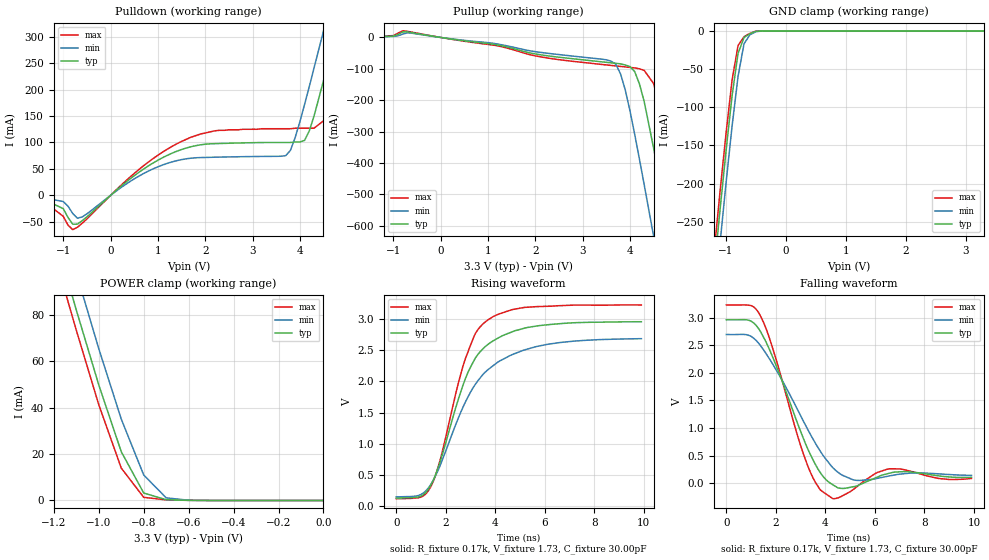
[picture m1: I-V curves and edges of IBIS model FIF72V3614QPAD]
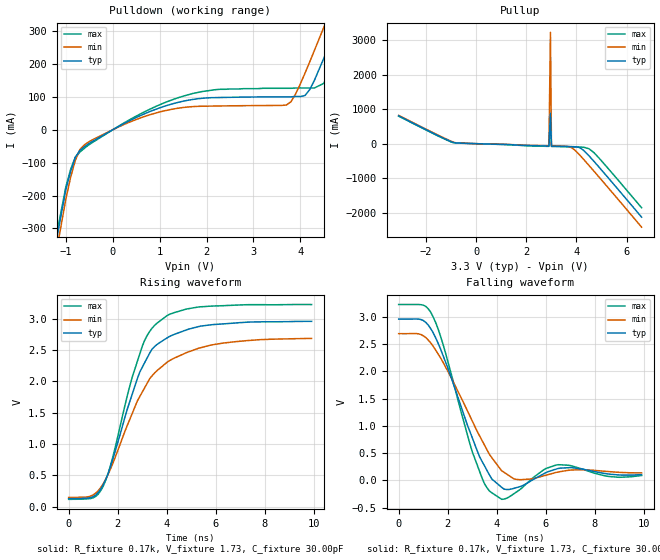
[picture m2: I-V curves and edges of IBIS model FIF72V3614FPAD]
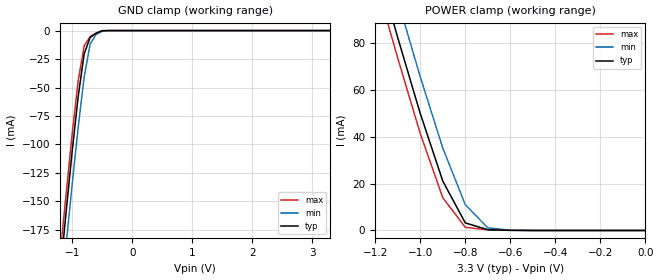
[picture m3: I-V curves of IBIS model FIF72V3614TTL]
| IBIS file i72v3612.ibs created by s2ibis2 version 1.1
| North Carolina State University Electronics Research Laboratory  1995
[IBIS ver]   2.1
[File name]   i72v3612.ibs
[File Rev]   1.0
[Date]   05/01/98
[Source]   Integrated Device Technology, Inc.
[Notes]   1. Temperatures: typ=25C, min=70C, max=0C 2. Cemos8_3.3V
   process. 3. Ramp rates based on 50 ohm load.
[Copyright]   Copyright 1997, Integrated Device Technology, Inc.
|   Component idt72V3612
[Component]   idt72V3612
[Manufacturer]   Integrated Device Technology
[Package]
| variable   typ   min   max
R_pkg   0.75   0.60   0.90
L_pkg   8.10nH   8.30nH   9.90nH
C_pkg   0.53pF   0.46pF   0.60pF
[Pin]  signal_name   model_name   R_pin   L_pin   C_pin
1   A23   FIF72V3614QPAD
2   A22   FIF72V3614QPAD
3   A21   FIF72V3614QPAD
4   GND   GND
5   A20   FIF72V3614QPAD
6   A19   FIF72V3614QPAD
7   A18   FIF72V3614QPAD
8   A17   FIF72V3614QPAD
9   A16   FIF72V3614QPAD
10   A15   FIF72V3614QPAD
11   A14   FIF72V3614QPAD
12   A13   FIF72V3614QPAD
13   A12   FIF72V3614QPAD
14   A11   FIF72V3614QPAD
15   A10   FIF72V3614QPAD
16   GND   GND
17   A9   FIF72V3614QPAD
18   A8   FIF72V3614QPAD
19   A7   FIF72V3614QPAD
20   VCC   POWER
21   A6   FIF72V3614QPAD
22   A5   FIF72V3614QPAD
23   A4   FIF72V3614QPAD
24   A3   FIF72V3614QPAD
25   GND   GND
26   A2   FIF72V3614QPAD
27   A1   FIF72V3614QPAD
28   A0   FIF72V3614QPAD
29   EFAL   FIF72V3614FPAD
30   AEAL   FIF72V3614FPAD
31   AFAL   FIF72V3614FPAD
32   FFAL   FIF72V3614FPAD
33   CSAL   FIF72V3614TTL
34   ENA   FIF72V3614TTL
35   CLKA   FIF72V3614TTL
36   W_RA   FIF72V3614TTL
37   VCC   POWER
38   PGA   FIF72V3614TTL
39   PEFAL   FIF72V3614FPAD
40   MBF2   FIF72V3614FPAD
41   MBA   FIF72V3614TTL
42   FS1   FIF72V3614TTL
43   FS0   FIF72V3614TTL
44   ODD_EVEN   FIF72V3614TTL
45   RST   FIF72V3614TTL
46   GND   GND
47   NC   NC
48   NC   NC
49   NC   NC
50   NC   NC
51   MBB   FIF72V3614TTL
52   MBF1   FIF72V3614FPAD
53   PEFBL   FIF72V3614FPAD
54   PGB   FIF72V3614TTL
55   VCC   POWER
56   W_RB   FIF72V3614TTL
57   CLKB   FIF72V3614TTL
58   ENB   FIF72V3614TTL
59   CSBL   FIF72V3614TTL
60   FFBL   FIF72V3614FPAD
61   AFBL   FIF72V3614FPAD
62   AEBL   FIF72V3614FPAD
63   EFBL   FIF72V3614FPAD
64   B0   FIF72V3614QPAD
65   B1   FIF72V3614QPAD
66   B2   FIF72V3614QPAD
67   GND   GND
68   B3   FIF72V3614QPAD
69   B4   FIF72V3614QPAD
70   B5   FIF72V3614QPAD
71   B6   FIF72V3614QPAD
72   VCC   POWER
73   B7   FIF72V3614QPAD
74   B8   FIF72V3614QPAD
75   B9   FIF72V3614QPAD
76   GND   GND
77   B10   FIF72V3614QPAD
78   B11   FIF72V3614QPAD
79   B12   FIF72V3614QPAD
80   B13   FIF72V3614QPAD
81   B14   FIF72V3614QPAD
82   B15   FIF72V3614QPAD
83   B16   FIF72V3614QPAD
84   B17   FIF72V3614QPAD
85   B18   FIF72V3614QPAD
86   B19   FIF72V3614QPAD
87   B20   FIF72V3614QPAD
88   GND   GND
89   B21   FIF72V3614QPAD
90   B22   FIF72V3614QPAD
91   B23   FIF72V3614QPAD
92   B24   FIF72V3614QPAD
93   B25   FIF72V3614QPAD
94   B26   FIF72V3614QPAD
95   VCC   POWER
96   B27   FIF72V3614QPAD
97   B28   FIF72V3614QPAD
98   B29   FIF72V3614QPAD
99   GND   GND
100   B30   FIF72V3614QPAD
101   B31   FIF72V3614QPAD
102   B32   FIF72V3614QPAD
103   B33   FIF72V3614QPAD
104   B34   FIF72V3614QPAD
105   B35   FIF72V3614QPAD
106   GND   GND
107   A35   FIF72V3614QPAD
108   A34   FIF72V3614QPAD
109   A33   FIF72V3614QPAD
110   A32   FIF72V3614QPAD
111   A31   FIF72V3614QPAD
112   A30   FIF72V3614QPAD
113   GND   GND
114   A29   FIF72V3614QPAD
115   A28   FIF72V3614QPAD
116   A27   FIF72V3614QPAD
117   VCC   POWER
118   A26   FIF72V3614QPAD
119   A25   FIF72V3614QPAD
120   A24   FIF72V3614QPAD
| Models and submodels in the file (3): FIF72V3614QPAD (I/O), FIF72V3614FPAD (Output), FIF72V3614TTL (Input)
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| FIN  FIN   dummy_model
| QIN  QIN   dummy_model
| QOEL QOEL   dummy_model
|   Model FIF72V3614QPAD
[Model]   FIF72V3614QPAD
Model_type   I/O
Polarity   Non-Inverting
Enable   Active-Low
Vinl =  0.800V
Vinh =  2.000V
Vmeas =  1.500V
C_comp   3.00pF   NA   NA
[Temperature Range]   25.00   70.00   0.000
[Voltage Range]   3.30V   3.00V   3.60V
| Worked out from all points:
|   slope of the pulldown table from 0 to 0.495 V, typ, clamps not added: 13.5 ohm
|   slope of the pullup table from 0 to 0.495 V, typ, clamps not added: 46.5 ohm
|   GND clamp passes 1 mA (typ) near -0.52 V on its own axis
|   POWER clamp passes 1 mA (typ) near -0.72 V on its own axis
|   rising waveform, R_fixture 0.17k, V_fixture 1.73, C_fixture 30.00pF: 20-80 % time 1.47ns typ, 1.9ns min, 1.25ns max; typ from 0.128 V to 2.96 V
|   falling waveform, R_fixture 0.17k, V_fixture 1.73, C_fixture 30.00pF: 20-80 % time 1.46ns typ, 1.86ns min, 1.22ns max; typ from 2.96 V to 0.105 V
[Pulldown]
| voltage   I(typ)   I(min)   I(max)
-3.3V     -1mA       -1mA       -1mA
-1.5V     -4.2mA     -3.2mA     -5mA
-800mV    -54.6mA    -34.52mA   -64.94mA
-600mV    -47.99mA   -40.8mA    -52.81mA
600mV     43.67mA    36.44mA    48.95mA
1.5V      86.71mA    67.57mA    102mA
3.7V      100mA      75.02mA    126mA
4.1V      104mA      172mA      127mA
4.5V      217mA      311mA      141mA
4.7V      287mA      383mA      200mA
5.1V      430mA      528mA      340mA
6.6V      980mA      1.077A     888mA
[Pullup]
| voltage   I(typ)   I(min)   I(max)
-3.3V     300uA      300uA      300uA
-800mV    17.75mA    10.87mA    21.29mA
3.6V      -80.87mA   -75.44mA   -89.18mA
3.9V      -87.82mA   -167mA     -93.93mA
4.1V      -109mA     -309mA     -97.12mA
4.3V      -204mA     -469mA     -105mA
4.5V      -353mA     -634mA     -147mA
4.7V      -515mA     -801mA     -262mA
4.9V      -682mA     -970mA     -418mA
5.1V      -851mA     -1.14A     -583mA
5.3V      -1.02A     -1.31A     -751mA
6.6V      -2.136A    -2.428A    -1.864A
[GND_clamp]
| voltage   I(typ)   I(min)   I(max)
-3.3V     -2.102A    -2.142A    -2.08A
-1.2V     -314mA     -358mA     -291mA
-1.1V     -234mA     -278mA     -210mA
-1V       -157mA     -199mA     -134mA
-900mV    -85.1mA    -125mA     -64.47mA
-800mV    -29.4mA    -59.48mA   -19.05mA
-700mV    -8.491mA   -16.63mA   -7.437mA
-600mV    -3.454mA   -4.697mA   -2.961mA
-500mV    -293uA     -833uA     -94.53uA
-400mV    -15.41nA   -678nA     -4.678nA
3.3V      33nA       34.31nA    33nA
[POWER_clamp]
| voltage   I(typ)   I(min)   I(max)
-3.3V     879mA      893mA      871mA
-1.2V     116mA      132mA      107mA
-1.1V     82.2mA     98.22mA    73.49mA
-1V       49.87mA    65.51mA    41.33mA
-900mV    21.08mA    35.16mA    13.99mA
-800mV    3.228mA    11mA       1.36mA
-700mV    330uA      1.138mA    265uA
-600mV    63.58uA    105uA      57uA
0V        33nA       30nA       36nA
[Ramp]
| variable   typ   min   max
dV/dt_r   1.06/0.84n   0.90/0.96n   1.22/0.77n
dV/dt_f   1.54/1.40n   1.33/1.99n   1.73/1.11n
R_load = 50.00
[Rising Waveform]
R_fixture = 0.17k
V_fixture = 1.73
C_fixture = 30.00pF
R_dut = 0.75
L_dut = 8.10nH
C_dut = 0.53pF
| time   V(typ)   V(min)   V(max)
0s        128mV      147mV      118mV
1ns       159mV      186mV      143mV
1.4ns     338mV      348mV      314mV
1.8ns     744mV      677mV      775mV
2.8ns     2.051V     1.675V     2.373V
3.2ns     2.379V     1.956V     2.772V
3.6ns     2.561V     2.151V     2.956V
4.7ns     2.799V     2.433V     3.154V
5.7ns     2.891V     2.563V     3.201V
9.9ns     2.958V     2.686V     3.227V
[Falling Waveform]
R_fixture = 0.17k
V_fixture = 1.73
C_fixture = 30.00pF
R_dut = 0.75
L_dut = 8.10nH
C_dut = 0.53pF
| time   V(typ)   V(min)   V(max)
0s        2.959V     2.692V     3.227V
1ns       2.935V     2.659V     3.215V
1.4ns     2.729V     2.479V     3.009V
1.9ns     2.253V     2.136V     2.402V
3.1ns     823mV      1.134V     545mV
3.9ns     124mV      505mV      -158mV
4.4ns     -56.7mV    237mV      -280mV
5.2ns     -59.1mV    52.64mV    -89.82mV
6.6ns     181mV      132mV      260mV
9.9ns     105mV      140mV      85.54mV
|   Model FIF72V3614FPAD
[Model]   FIF72V3614FPAD
Model_type   Output
Vmeas =  1.500V
C_comp   3.00pF   NA   NA
[Temperature Range]   25.00   70.00   0.000
[Voltage Range]   3.30V   3.00V   3.60V
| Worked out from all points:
|   slope of the pulldown table from 0 to 0.495 V, typ, clamps not added: 13.5 ohm
|   slope of the pullup table from 0 to 0.495 V, typ, clamps not added: 46.5 ohm
|   rising waveform, R_fixture 0.17k, V_fixture 1.73, C_fixture 30.00pF: 20-80 % time 1.47ns typ, 1.86ns min, 1.28ns max; typ from 0.128 V to 2.96 V
|   falling waveform, R_fixture 0.17k, V_fixture 1.73, C_fixture 30.00pF: 20-80 % time 1.36ns typ, 1.7ns min, 1.14ns max; typ from 2.96 V to 0.104 V
[Pulldown]
| voltage   I(typ)   I(min)   I(max)
-3.3V     -2.095A    -2.135A    -2.074A
-1.5V     -565mA     -607mA     -542mA
-1V       -181mA     -210mA     -173mA
-700mV    -62.83mA   -59.84mA   -67.64mA
500mV     37.14mA    31.18mA    41.46mA
1.9V      95.58mA    71.46mA    116mA
3.7V      100mA      75.02mA    126mA
4.1V      104mA      172mA      127mA
4.5V      217mA      311mA      141mA
4.7V      287mA      383mA      200mA
5.1V      430mA      528mA      340mA
6.6V      980mA      1.077A     888mA
[Pullup]
| voltage   I(typ)   I(min)   I(max)
-3.1V     805mA      820mA      797mA
-1.5V     223mA      238mA      214mA
-1V       54.39mA    68.64mA    47.35mA
-800mV    20.98mA    21.87mA    22.65mA
2.9V      -69.66mA   -61.22mA   -77.9mA
2.96V     879mA      3.227A     871mA
3V        -71.29mA   -62.83mA   -79.53mA
3.8V      -84.18mA   -116mA     -92.35mA
4.1V      -108mA     -308mA     -97.12mA
4.5V      -352mA     -632mA     -147mA
4.9V      -680mA     -967mA     -417mA
6.6V      -2.129A    -2.419A    -1.857A
[Ramp]
| variable   typ   min   max
dV/dt_r   1.06/0.84n   0.90/0.98n   1.22/0.78n
dV/dt_f   1.54/1.26n   1.34/1.63n   1.73/1.06n
R_load = 50.00
[Rising Waveform]
R_fixture = 0.17k
V_fixture = 1.73
C_fixture = 30.00pF
R_dut = 0.75
L_dut = 8.10nH
C_dut = 0.53pF
| time   V(typ)   V(min)   V(max)
0s        128mV      147mV      118mV
1ns       160mV      189mV      143mV
1.4ns     344mV      360mV      321mV
1.7ns     634mV      598mV      651mV
2.5ns     1.69V      1.403V     1.941V
3ns       2.226V     1.831V     2.562V
3.6ns     2.59V      2.172V     2.93V
4.3ns     2.75V      2.371V     3.098V
5.8ns     2.904V     2.581V     3.202V
9.9ns     2.959V     2.687V     3.227V
[Falling Waveform]
R_fixture = 0.17k
V_fixture = 1.73
C_fixture = 30.00pF
R_dut = 0.75
L_dut = 8.10nH
C_dut = 0.53pF
| time   V(typ)   V(min)   V(max)
0s        2.959V     2.692V     3.227V
900ps     2.952V     2.677V     3.224V
1.4ns     2.713V     2.464V     3.003V
1.8ns     2.3V       2.173V     2.508V
3ns       779mV      1.087V     522mV
3.5ns     263mV      643mV      -66.12mV
3.8ns     21.74mV    413mV      -231mV
4.7ns     -148mV     25.59mV    -246mV
6.5ns     217mV      152mV      286mV
9.9ns     104mV      136mV      87.61mV
|   Model FIF72V3614TTL
[Model]   FIF72V3614TTL
Model_type   Input
Vinl =  0.800V
Vinh =  2.000V
Vmeas =  1.500V
C_comp   3.00pF   NA   NA
[Temperature Range]   25.00   70.00   0.000
[Voltage Range]   3.30V   3.00V   3.60V
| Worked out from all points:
|   GND clamp passes 1 mA (typ) near -0.54 V on its own axis
|   POWER clamp passes 1 mA (typ) near -0.72 V on its own axis
[GND_clamp]
| voltage   I(typ)   I(min)   I(max)
-3.3V     -1.418A    -1.445A    -1.403A
-1.2V     -213mA     -242mA     -197mA
-1.1V     -159mA     -188mA     -143mA
-1V       -106mA     -135mA     -90.74mA
-900mV    -58.01mA   -85.04mA   -44.07mA
-800mV    -20.35mA   -40.72mA   -13.32mA
-700mV    -5.991mA   -11.62mA   -5.227mA
-600mV    -2.408mA   -3.311mA   -2.038mA
-500mV    -184uA     -573uA     -45.85uA
-400mV    -12.08nA   -481nA     -4.48nA
3.3V      33nA       34.31nA    33nA
[POWER_clamp]
| voltage   I(typ)   I(min)   I(max)
-3.3V     879mA      893mA      871mA
-1.2V     116mA      132mA      107mA
-1.1V     82.2mA     98.22mA    73.49mA
-1V       49.87mA    65.51mA    41.33mA
-900mV    21.08mA    35.16mA    13.99mA
-800mV    3.228mA    11mA       1.36mA
-700mV    330uA      1.138mA    265uA
-600mV    63.58uA    105uA      57uA
0V        33nA       30nA       36nA
